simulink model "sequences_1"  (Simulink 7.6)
settings: Solver=ode15s  StartTime=0.0  StopTime=2/60  FixedStep=Ts  RelTol=1e-3
InitFcn:
  | clc
  | a=exp(j*2*pi/3);
  | Ts=5e-5;
undefined symbols (not defined in the file or in its folder): Angle, Magnitude
libraries: powerlib x9, powerlib_extras x3

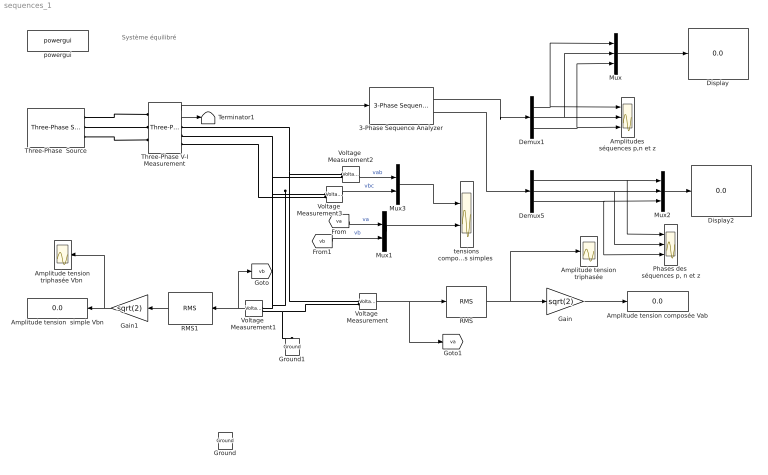
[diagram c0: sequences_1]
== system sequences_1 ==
  note: Système équilibré
  3-Phase Sequence Analyzer : powerlib_extras/Measurements/3-Phase Sequence Analyzer  DialogController=POWERSYS.PowerSysDialog  SystemSampleTime=-1  f1=60  n=1  seq=Positive Negative Zero
  Amplitude tension  simple Vbn : Display
  Amplitude tension composée Vab : Display
  Amplitude tension triphasée : Scope
  "Amplitude tension triphasée Vbn " : Scope
  Amplitudes séquences p,n et z : Scope  NumInputPorts=3
  Demux1 : Demux  Outputs=3
  Demux5 : Demux  Outputs=3
  Display : Display
  Display2 : Display
  Gain : Gain  Gain=sqrt(2)
  Gain1 : Gain  Gain=sqrt(2)
  Ground : powerlib/Elements/Ground  DialogController=POWERSYS.PowerSysDialog  PhysicalDomain=powersysdomain  SubClassName=unknown  LeftPortType=p1  RightPortType=p1  LConnTagsString=a
  Ground1 : powerlib/Elements/Ground  DialogController=POWERSYS.PowerSysDialog  PhysicalDomain=powersysdomain  SubClassName=unknown  LeftPortType=p1  RightPortType=p1  LConnTagsString=a
  Mux : Mux  Inputs=3
  Mux1 : Mux  Inputs=2
  Mux2 : Mux  Inputs=3
  Mux3 : Mux  Inputs=2
  "Phases des  séquences p, n et z" : Scope  NumInputPorts=3
  RMS : powerlib_extras/Measurements/RMS  DialogController=POWERSYS.PowerSysDialog  SystemSampleTime=-1  f1=60
  RMS1 : powerlib_extras/Measurements/RMS  DialogController=POWERSYS.PowerSysDialog  SystemSampleTime=-1  f1=60
  Terminator1 : Terminator
  Three-Phase V-I Measurement : powerlib/Measurements/Three-Phase V-I Measurement  DialogController=POWERSYS.PowerSysDialog  SystemSampleTime=-1  VoltageMeasurement=phase-to-ground  SetLabelV=off  LabelV=Vabc  Vpu=off  VpuLL=off  CurrentMeasurement=yes  SetLabelI=off  LabelI=Iabc  Ipu=off  Pbase=100e6  Vbase=500e3  OutputType=Magnitude-Angle  PhasorSimulation=off  PSBequivalent=0
  Three-Phase  Source : powerlib/Electrical Sources/Three-Phase Source  DialogController=POWERSYS.PowerSysDialog  SystemSampleTime=-1  Voltage=220*sqrt(3)/sqrt(2)  PhaseAngle=0  Frequency=60  InternalConnection=Yg  SpecifyImpedance=off  Resistance=0.8929  Inductance=1e-6  ShortCircuitLevel=100e6  BaseVoltage=25e3  XRratio=1e-12
  Voltage  Measurement{,1..3} (4 alike) : powerlib/Measurements/Voltage Measurement  DialogController=POWERSYS.PowerSysDialog  SystemSampleTime=-1  PhasorSimulation=off  OutputType=Complex  PSBequivalent=0
  powergui : powerlib/powergui  Priority=1  SystemSampleTime=-1  SimulationMode=Continuous  SampleTime=Ts  frequency=60  SPID=off  DisableSnubberDevices=off  DisableRonSwitches=off  DisableVfSwitches=off  SwTol=0  Interpol=off  frequencyindice=60  echomessages=off  HookPort=off  DisplayEquations=off  FunctionMessages=off  EnableUseOfTLC=off  x0status=blocks  RestoreLinks=warning  ResistiveCurrentMeasurement=off  Ylog=off  Xlog=on  ShowGrid=off  save=off  variable=ZData  ZoomFFT=off  StartTime=0.0  cycles=1  DisplayStyle=1  FreqAxis=off  MaxFrequency=1000  frequencyindicesteady=1  display=off  methode=off
  "tensions composées  et tensions simples " : Scope  NumInputPorts=2
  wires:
  Three-Phase V-I Measurement/2 -> Terminator1/1
  Three-Phase V-I Measurement/1 -> 3-Phase Sequence Analyzer/1
  3-Phase Sequence Analyzer/1 -> Demux1/1
  Demux1/1 -> Amplitudes séquences p,n et z/1, Mux/1
  Demux1/2 -> Amplitudes séquences p,n et z/2, Mux/2
  Demux1/3 -> Amplitudes séquences p,n et z/3, Mux/3
  Mux/1 -> Display/1
  Mux2/1 -> Display2/1
  Demux5/1 -> Mux2/1, "Phases des  séquences p, n et z"/1
  Demux5/2 -> Mux2/2, "Phases des  séquences p, n et z"/2
  Demux5/3 -> Mux2/3, "Phases des  séquences p, n et z"/3
  3-Phase Sequence Analyzer/2 -> Demux5/1
  Voltage  Measurement/1 -> RMS/1, [va]
  RMS/1 -> Gain/1, Amplitude tension triphasée/1
  Gain/1 -> Amplitude tension composée Vab/1
  Voltage  Measurement1/1 -> RMS1/1, [vb]
  RMS1/1 -> Gain1/1
  Gain1/1 -> Amplitude tension  simple Vbn/1, "Amplitude tension triphasée Vbn "/1
  [va] -> Mux1/1  "va"
  [vb] -> Mux1/2  "vb"
  Voltage  Measurement3/1 -> Mux3/2  "vbc"
  Voltage  Measurement2/1 -> Mux3/1  "vab"
  Mux3/1 -> "tensions composées  et tensions simples "/1
  Mux1/1 -> "tensions composées  et tensions simples "/2
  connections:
  Three-Phase V-I Measurement/RConn1 -- Voltage  Measurement/LConn1 -- Voltage  Measurement2/LConn1
  Voltage  Measurement1/LConn1 -- Voltage  Measurement3/LConn1 -- Three-Phase V-I Measurement/RConn2 -- Voltage  Measurement2/LConn2
  Voltage  Measurement1/LConn2 -- Ground1/LConn1 -- Voltage  Measurement/LConn2
  Three-Phase V-I Measurement/RConn3 -- Voltage  Measurement3/LConn2
  Three-Phase  Source/RConn1 -- Three-Phase V-I Measurement/LConn1
  Three-Phase  Source/RConn2 -- Three-Phase V-I Measurement/LConn2
  Three-Phase  Source/RConn3 -- Three-Phase V-I Measurement/LConn3
